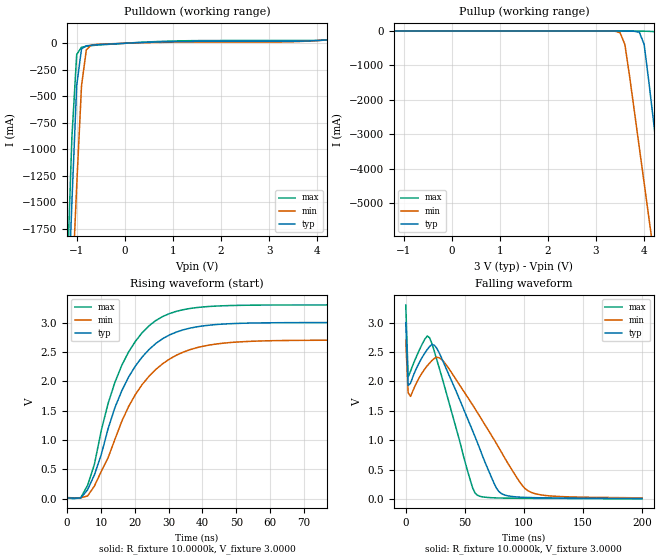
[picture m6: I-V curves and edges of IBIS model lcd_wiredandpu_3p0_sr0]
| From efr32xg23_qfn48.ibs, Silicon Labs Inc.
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|   Model lcd_wiredandpu_3p0_sr0
[Model]  lcd_wiredandpu_3p0_sr0
Model_type Output
Polarity   Inverting
Enable   Active-Low
C_comp   1.6300pF   1.4000pF   2.7000pF
[Temperature Range]   25.0000   0.1250k   -40.0000
[Pullup Reference]   3.0000V   2.7000V   3.3000V
[Pulldown Reference]   0.0V   0.0V   0.0V
[POWER Clamp Reference]   3.0000V   2.7000V   3.3000V
[GND Clamp Reference]   0.0V   0.0V   0.0V
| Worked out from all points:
|   slope of the pulldown table from 0 to 0.45 V, typ, clamps not added: 50.8 ohm
|   slope of the pullup table from 0 to 0.45 V, typ, clamps not added: 40.2 kohm
|   rising waveform, R_fixture 10.0000k, V_fixture 3.0000: 20-80 % time 12.8ns typ, 14.7ns min, 11.4ns max; typ from 0.013 V to 3 V
|   falling waveform, R_fixture 10.0000k, V_fixture 3.0000: 20-80 % time 37.3ns typ, 49.8ns min, 27.6ns max; typ from 3 V to 0.013 V
[Pulldown]
|Voltage   I(typ)   I(min)   I(max)
-3V       -24.29A    -21.98A    -26.6A
-1.2V     -2.696A    -3.401A    -2.229A
-1.1V     -1.504A    -2.372A    -891.2mA
-1V       -398.3mA   -1.347A    -105.5mA
-900mV    -52.43mA   -401.6mA   -36.73mA
-800mV    -23.94mA   -62.62mA   -28.56mA
-700mV    -18.26mA   -17.6mA    -22.48mA
1.1V      16.3mA     10.6mA     22.34mA
3.3V      18.98mA    12.76mA    25.98mA
4.1V      28.82mA    28.1mA     28.94mA
4.9V      58.93mA    54.83mA    59.76mA
6V        113.9mA    103.8mA    120.1mA
[Pullup]
|Voltage   I(typ)   I(min)   I(max)
-3V       74.15uA    73.25uA    86.28uA
3.5V      -515.4uA   -50.46mA   -100.7uA
3.6V      -1.645mA   -390.8mA   -104.2uA
4V        -385.9mA   -4.417A    -4.327mA
4.1V      -1.495A    -5.447A    -8.512mA
4.2V      -2.686A    -6.476A    -15.06mA
4.3V      -3.882A    -7.507A    -84.3mA
4.4V      -5.077A    -8.538A    -881.9mA
4.5V      -6.274A    -9.569A    -2.22A
4.7V      -8.669A    -11.63A    -4.917A
4.8V      -9.868A    -12.66A    -6.266A
6V        -24.27A    -25.05A    -22.51A
[Ramp]
| variable   typ   min   max
dV/dt_r  0.3580/12.9871n   0.2880/14.5925n   0.4423/11.6890n
dV/dt_f  1.7920/66.4020n   1.6058/86.8761n   1.9738/48.6868n
R_load = 10.0000k
[Rising Waveform]
R_fixture= 10.0000k
V_fixture= 3.0000
V_fixture_min= 2.7000
V_fixture_max= 3.3000
|time   V(typ)   V(min)   V(max)
0s        12.55mV    17.32mV    10.21mV
4.04ns    10.23mV    14.7mV     13.88mV
6.061ns   149.7mV    44.66mV    225.4mV
8.081ns   404.1mV    213.5mV    584.2mV
12.12ns   1.19V      696.2mV    1.621V
18.18ns   2.072V     1.569V     2.499V
24.24ns   2.542V     2.086V     2.946V
32.32ns   2.838V     2.444V     3.191V
58.59ns   2.995V     2.688V     3.298V
200ns     3V         2.7V       3.3V
[Falling Waveform]
R_fixture= 10.0000k
V_fixture= 3.0000
V_fixture_min= 2.7000
V_fixture_max= 3.3000
|time   V(typ)   V(min)   V(max)
0s        3V         2.7V       3.3V
2.02ns    1.933V     1.808V     2.077V
16.16ns   2.483V     2.213V     2.719V
20.2ns    2.595V     2.314V     2.741V
30.3ns    2.4V       2.375V     2.095V
54.55ns   1.263V     1.666V     331.3mV
60.61ns   967.4mV    1.475V     70.17mV
78.79ns   133.7mV    878.3mV    22.41mV
105.1ns   29.91mV    128.1mV    16.07mV
200ns     13.3mV     23.61mV    10.3mV
